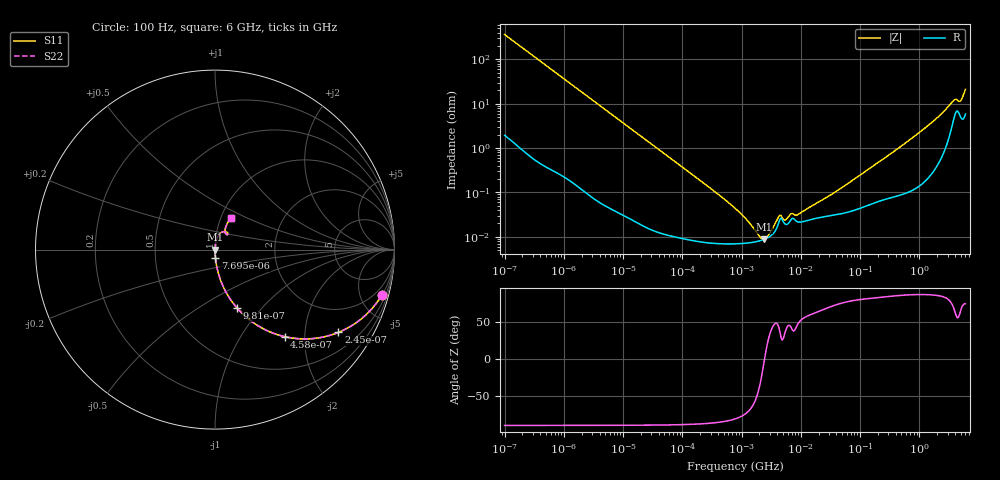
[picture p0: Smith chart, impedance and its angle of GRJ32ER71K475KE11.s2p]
!Murata Part Number: GRJ32ER71K475KE11
!These Parameters are Measured in Series Mode Connection
!Data Generated on Jun 19, 2026
!  o--ll--o
!Port1  Port2
!  o------o
!Operation Temp=25[degC], DC Bias Voltage=0[V]
!Freq. Start=100[Hz] Stop=6[GHz] 401[Steps]
# Hz S RI R 50
!Freq.(Hz) S11(Real) S11(Imag) S21(Real) S21(Imag) S12(Real) S12(Imag) S22(Real) S22(Imag)
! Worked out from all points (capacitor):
!   401 points, 100 Hz to 6 GHz, reference 50 ohm
!   read as one part in series: C = 4.38 uF near 109 Hz
!   lowest |Z| = 8.74 mohm at 2.373 MHz (marker M1)
!   series resonance near 2.447 MHz, so ESL is about 970 pH
!   S11 on the Smith chart (normalised r, x): 100 Hz: 1.04, -7.26; 245 Hz: 1.01, -2.97; 458 Hz: 1.01, -1.59; 981 Hz: 1.00, -0.74; 7.695 kHz: 1.00, -0.10; 6 GHz: 1.12, +0.41
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100  0.9282 -0.2555  0.0718 0.2555  0.0718 0.2555  0.9282 -0.2555
245  0.6876 -0.4611  0.3124 0.4611  0.3124 0.4611  0.6876 -0.4611
458  0.388 -0.4848  0.612 0.4848  0.612 0.4848  0.388 -0.4848
981  0.1234 -0.3258  0.8766 0.3258  0.8766 0.3258  0.1234 -0.3258
2008  0.0333 -0.1763  0.9667 0.1763  0.9667 0.1763  0.0333 -0.1763
7695  0.00265 -0.0477  0.9974 0.0477  0.9974 0.0477  0.00265 -0.0477
40335  0.000208 -0.00919  0.9998 0.00919  0.9998 0.00919  0.000208 -0.00919
774597  6.95e-05 -0.000436  0.9999 0.000436  0.9999 0.000436  6.95e-05 -0.000436
1212075  7.19e-05 -0.000234  0.9999 0.000234  0.9999 0.000234  7.19e-05 -0.000234
1896632  7.93e-05 -8e-05  0.9999 8e-05  0.9999 8e-05  7.93e-05 -8e-05
2372521  8.69e-05 -9.7e-06  0.9999 9.7e-06  0.9999 9.7e-06  8.69e-05 -9.7e-06
2967816  0.000101 6.31e-05  0.9999 -6.31e-05  0.9999 -6.31e-05  0.000101 6.31e-05
4246196  0.00021 0.000194  0.9998 -0.000194  0.9998 -0.000194  0.00021 0.000194
5554849  0.00019 0.000149  0.9998 -0.000149  0.9998 -0.000149  0.00019 0.000149
6948629  0.000251 0.000221  0.9997 -0.000221  0.9997 -0.000221  0.000251 0.000221
9090158  0.000215 0.000237  0.9998 -0.000237  0.9998 -0.000237  0.000215 0.000237
1.555665e7  0.000249 0.000435  0.9998 -0.000435  0.9998 -0.000435  0.000249 0.000435
3.124326e8  0.00079 0.00702  0.9992 -0.00702  0.9992 -0.00702  0.00079 0.00702
1.565993e9  0.00376 0.0359  0.9962 -0.0359  0.9962 -0.0359  0.00376 0.0359
3.666503e9  0.0451 0.0993  0.9549 -0.0993  0.9549 -0.0993  0.0451 0.0993
5.016141e9  0.0566 0.0963  0.9434 -0.0963  0.9434 -0.0963  0.0566 0.0963
6e9  0.0886 0.1747  0.9114 -0.1747  0.9114 -0.1747  0.0886 0.1747
